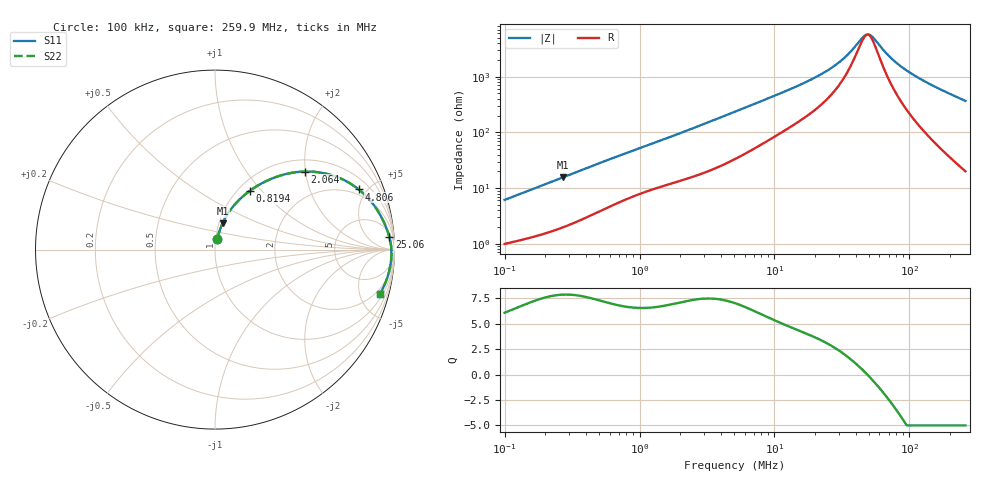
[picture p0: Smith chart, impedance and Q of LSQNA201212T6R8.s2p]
! LSQNA201212T6R8  S-PARAMETER MODEL  ( General Type )
! Model Generated by TAIYO YUDEN Corporation (http://www.ty-top.com)
! Version 3.0
! TAIYO YUDEN Control No. 110926NF25SB-FKC
! Copyright(c) 2007 TAIYO YUDEN CO.,LTD. All Rights Reserved.
! Product Description (link to TY-COMPAS)
! https://ds.yuden.co.jp/TYCOMPAS/or/detail?pn=LSQNA201212T6R8M&u=M
! Products Name : Inductors
! Characteristics :
!  Inductance : 6.8 uH , SRF(min) : 38 MHz , DC Resistance(max) : 0.611 Ohm
!  Rated Current : Saturation :250 mA , Temp Rise : 540 mA (40 degC)
!  Case Size : 2.0 x 1.25 / 0.079 x 0.049 [mm/inch] , Thickness : 1.25 / 0.049 [mm/inch]
!  (Conditions: Temperature = 25 degC , DC Bias Current/Voltage = 0A / 0V)
! External Node Assignments :
!  1  o---GGG---o  2
! GND o---------o GND
! Frequency Range : 0.1MHz  -  259.929867MHz  [ 402 STEP ]
# MHz S RI R 50
! Freq[MHz].  S11 Real  S11 Imag  S21 Real  S21 Imag  S12 Real  S12 Imag  S22 Real  S22 Imag
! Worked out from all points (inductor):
!   401 points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, 100 kHz to 259.9 MHz, reference 50 ohm
!   read as one part in series: L = 9.5 uH near 104 kHz
!   highest Q = 7.87 at 272.5 kHz (marker M1), where L = 9.15 uH
!   self-resonance near 48.77 MHz
!   S11 on the Smith chart (normalised r, x): 100 kHz: 1.02, +0.12; 819.4 kHz: 1.13, +0.86; 2.064 MHz: 1.28, +1.98; 4.806 MHz: 1.62, +4.42; 25.06 MHz: 9, +25; 259.9 MHz: 1.40, -7.36
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0.1  0.0134 0.0593  0.9866 -0.0593  0.9866 -0.0593  0.0134 0.0593
0.272517  0.0421 0.1471  0.9579 -0.1471  0.9579 -0.1471  0.0421 0.1471
0.37324  0.0659 0.1917  0.9341 -0.1917  0.9341 -0.1917  0.0659 0.1917
0.819359  0.1933 0.3268  0.8067 -0.3268  0.8067 -0.3268  0.1933 0.3268
1.393082  0.3489 0.4077  0.6511 -0.4077  0.6511 -0.4077  0.3489 0.4077
2.064047  0.4993 0.4349  0.5007 -0.4349  0.5007 -0.4349  0.4993 0.4349
2.998647  0.6491 0.4151  0.3509 -0.4151  0.3509 -0.4151  0.6491 0.4151
4.806364  0.8013 0.3351  0.1987 -0.3351  0.1987 -0.3351  0.8013 0.3351
5.098332  0.8158 0.323  0.1842 -0.323  0.1842 -0.323  0.8158 0.323
8.840321  0.9088 0.2129  0.0912 -0.2129  0.0912 -0.2129  0.9088 0.2129
19.02902  0.9625 0.0995  0.0375 -0.0995  0.0375 -0.0995  0.9625 0.0995
25.05743  0.972 0.0681  0.028 -0.0681  0.028 -0.0681  0.972 0.0681
32.99563  0.9783 0.0391  0.0217 -0.0391  0.0217 -0.0391  0.9783 0.0391
45.19087  0.9823 0.00761  0.0177 -0.00761  0.0177 -0.00761  0.9823 0.00761
48.88766  0.9829 -0.00024  0.0171 0.00024  0.0171 0.00024  0.9829 -0.00024
50.84796  0.9831 -0.00418  0.0169 0.00418  0.0169 0.00418  0.9831 -0.00418
53.93677  0.9833 -0.0101  0.0167 0.0101  0.0167 0.0101  0.9833 -0.0101
71.02397  0.9828 -0.0389  0.0172 0.0389  0.0172 0.0389  0.9828 -0.0389
88.1685  0.9808 -0.0635  0.0192 0.0635  0.0192 0.0635  0.9808 -0.0635
116.1003  0.9752 -0.0989  0.0248 0.0989  0.0248 0.0989  0.9752 -0.0989
172.0189  0.9584 -0.1612  0.0416 0.1612  0.0416 0.1612  0.9584 -0.1612
259.9299  0.9199 -0.2455  0.0801 0.2455  0.0801 0.2455  0.9199 -0.2455
